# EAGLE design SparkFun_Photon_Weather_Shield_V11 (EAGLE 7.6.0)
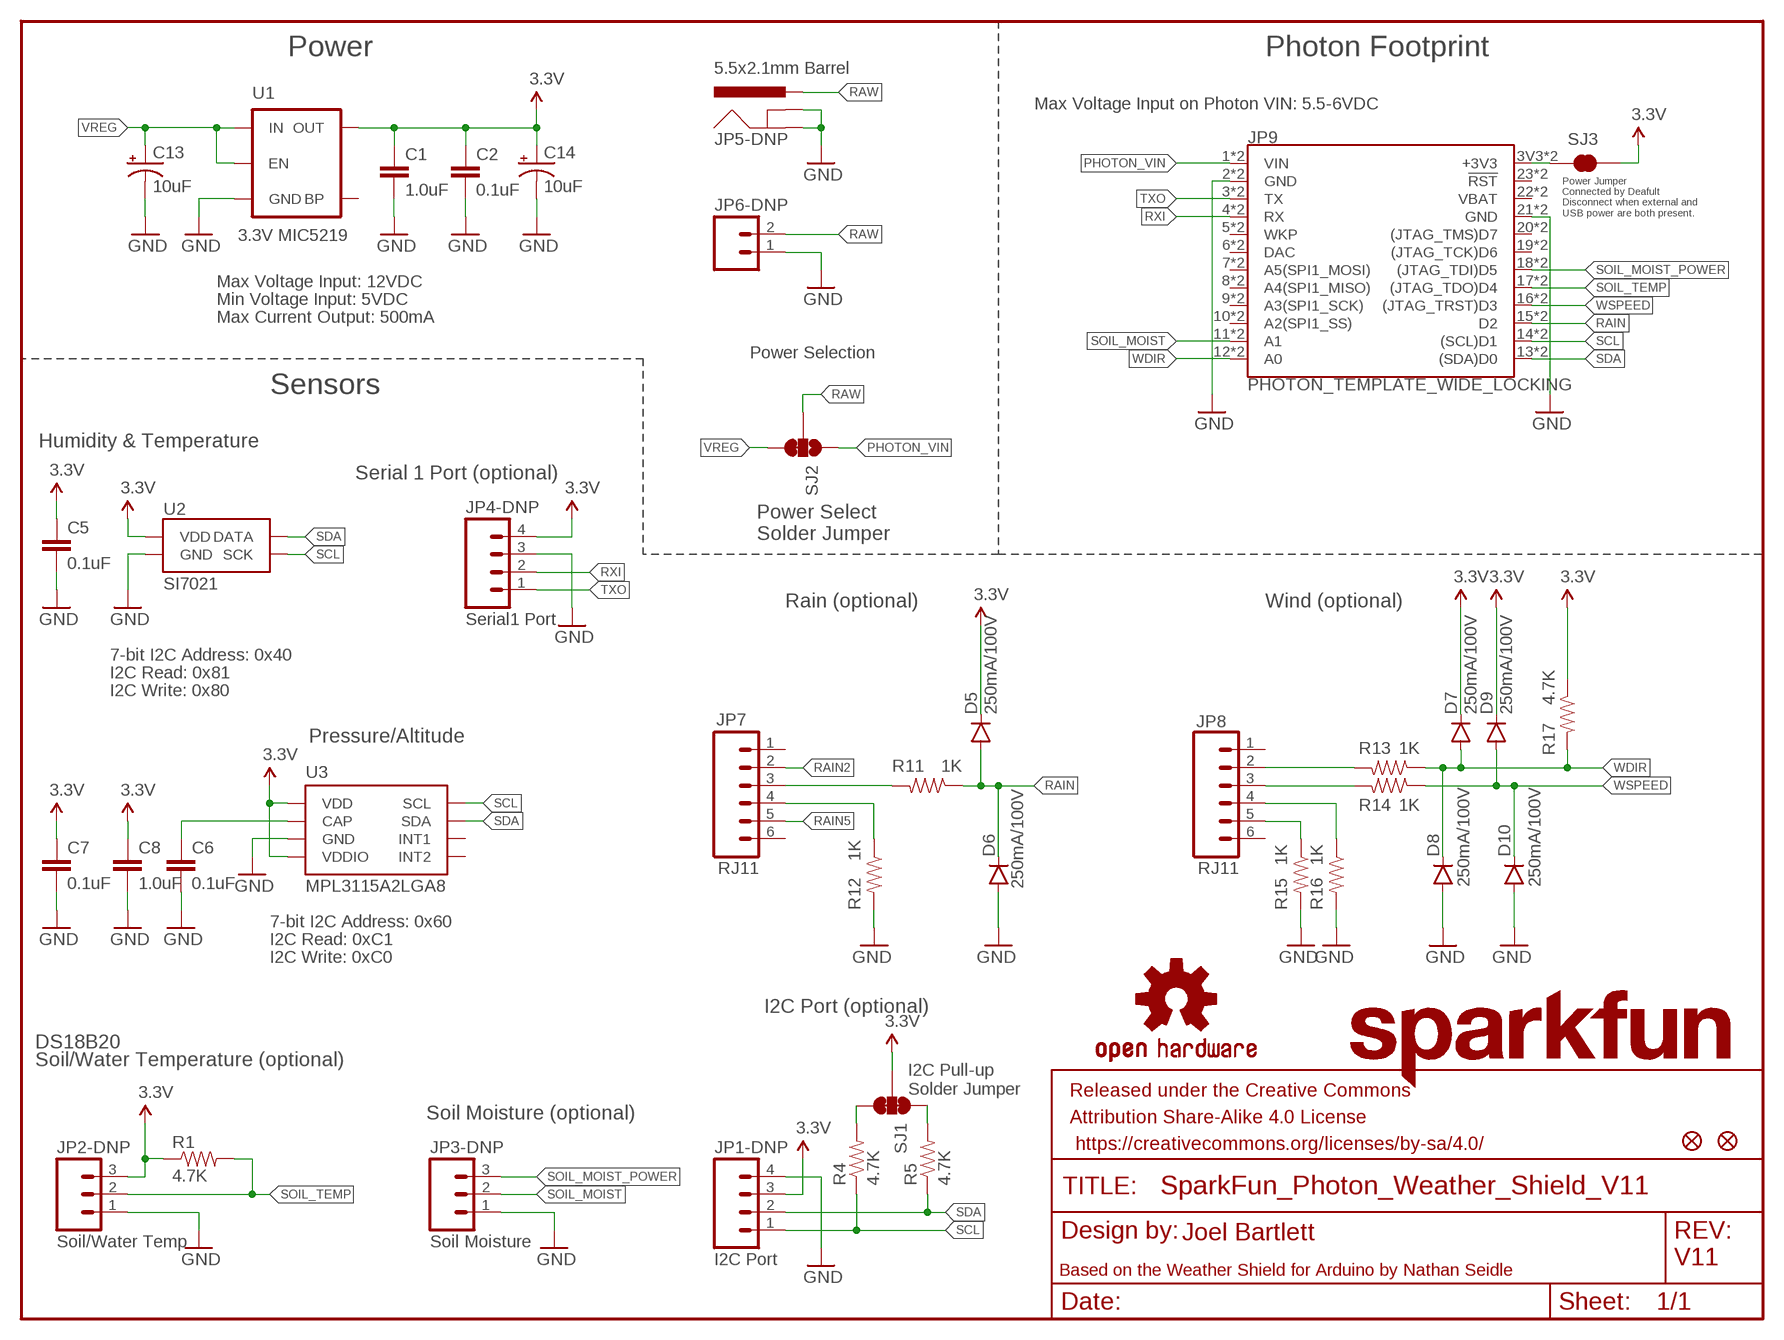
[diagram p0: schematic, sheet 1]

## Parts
C1  1.0uF  1.0UF-16V-10%(0603)  [0603-CAP]
C2  0.1uF  0.1UF-25V(+80/-20%)(0603)  [0603-CAP]
C5  0.1uF  0.1UF-25V(+80/-20%)(0603)  [0603-CAP]
C6  0.1uF  0.1UF-25V(+80/-20%)(0603)  [0603-CAP]
C7  0.1uF  0.1UF-25V(+80/-20%)(0603)  [0603-CAP]
C8  1.0uF  1.0UF-16V-10%(0603)  [0603-CAP]
C13  10uF  10UF-16V-10%(TANT)  [EIA3216]
C14  10uF  10UF-16V-10%(TANT)  [EIA3216]
D5  250mA/100V  DIODEBAS16  [SOD-323]
D6  250mA/100V  DIODEBAS16  [SOD-323]
D7  250mA/100V  DIODEBAS16  [SOD-323]
D8  250mA/100V  DIODEBAS16  [SOD-323]
D9  250mA/100V  DIODEBAS16  [SOD-323]
D10  250mA/100V  DIODEBAS16  [SOD-323]
FID1  FIDUCIAL1X2  [FIDUCIAL-1X2]
FID2  FIDUCIAL1X2  [FIDUCIAL-1X2]
FRAME1  FRAME-LETTER  [CREATIVE_COMMONS]
JP1-DNP  I2C Port  M04PTH  [1X04]
JP2-DNP  Soil/Water Temp  M03PTH  [1X03]
JP3-DNP  Soil Moisture  M03PTH  [1X03]
JP4-DNP  Serial1 Port  M04PTH  [1X04]
JP5-DNP  5.5x2.1mm Barrel  POWER_JACKSMD  [POWER_JACK_SMD]
JP6-DNP  M023.5MM  [SCREWTERMINAL-3.5MM-2]
JP7  RJ11  RJ11-6PTH  [RJ11-6]
JP8  RJ11  RJ11-6PTH  [RJ11-6]
JP9  PHOTON_TEMPLATE_WIDE_LOCKING  SPARK_PHOTONSPARK_PHOTON_TEMPLATE_WIDE_LOCKING  [SPARK_PHOTON_TEMPLATE_WIDE_LOCKING]
LOGO1  OSHW-LOGOM  [OSHW-LOGO-M]
LOGO2  SFE_LOGO_NAME.1_INCH  [SFE_LOGO_NAME_.1]
R1  4.7K  4.7KOHM-1/10W-1%(0603)  [0603-RES]
R4  4.7K  4.7KOHM-1/10W-1%(0603)  [0603-RES]
R5  4.7K  4.7KOHM-1/10W-1%(0603)  [0603-RES]
R11  1K  1KOHM-1/10W-1%(0603)  [0603-RES]
R12  1K  1KOHM-1/10W-1%(0603)  [0603-RES]
R13  1K  1KOHM-1/10W-1%(0603)  [0603-RES]
R14  1K  1KOHM-1/10W-1%(0603)  [0603-RES]
R15  1K  1KOHM-1/10W-1%(0603)  [0603-RES]
R16  1K  1KOHM-1/10W-1%(0603)  [0603-RES]
R17  4.7K  4.7KOHM-1/10W-1%(0603)  [0603-RES]
SJ1  JUMPER-PAD-3-NC_BY_TRACE  [PAD-JUMPER-3-3OF3_NC_BY_TRACE_YES_SILK_FULL_BOX]
SJ2  JUMPER-PAD-3-2OF3_NC_BY_TRACE_SMALL  [PAD-JUMPER-3-2OF3_NC_BY_TRACE_YES_SILK_FULL_BOX]
SJ3  JUMPER-PAD-2-NC_BY_TRACE  [PAD-JUMPER-2-NC_BY_TRACE_YES_SILK]
U1  3.3V MIC5219  MIC52053.3V  [SOT23-5]
U2  SI7021  [SI7021]
U3  MPL3115A2LGA8  [LGA8]

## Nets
3.3V: C1.1 C2.1 C5.1 C7.1 C8.1 C14.A(+) D5.C D7.C D9.C JP1-DNP.3 JP2-DNP.3 JP4-DNP.4 R1.1 R17.1 SJ1.2 SJ3.2 U1.5(OUT) U2.VDD U3.1(VDD) U3.4(VDDIO)
GND: C1.2 C2.2 C5.2 C6.2 C7.2 C8.2 C13.C(-) C14.C(-) D6.A D8.A D10.A JP1-DNP.4 JP2-DNP.1 JP3-DNP.1 JP4-DNP.3 JP5-DNP.GND(GNDBREAK) JP5-DNP.P$4(GND) JP6-DNP.1 JP9.2(GND) JP9.21(GND) JP9.GND@0(GND) JP9.GND@2(GND) R12.2 R15.2 R16.2 U1.2(GND) U2.GND U3.3(GND)
N$1: JP8.3 R14.2
N$2: JP8.2 R13.2
N$3: R4.2 SJ1.3
N$4: JP7.3 R11.2
N$5: C6.1 U3.2(CAP)
N$6: R5.2 SJ1.1
N$7: JP9.3V3(+3V3) JP9.24(+3V3) SJ3.1
N$11: JP7.4 R12.1
N$12: JP8.5 R15.1
N$13: JP8.4 R16.1
PHOTON_VIN: JP9.1(VIN) JP9.VIN SJ2.1
RAIN: D5.A D6.C JP9.15(D2) JP9.D2 R11.1
RAIN2: JP7.2
RAIN5: JP7.5
RAW [vcc]: JP5-DNP.VIN0(PWR) JP6-DNP.2 SJ2.2
RXI: JP4-DNP.2 JP9.4(RX) JP9.RX
SCL: JP1-DNP.1 JP9.14((SCL)D1) JP9.D1((SCL)D1) R4.1 U2.SCK U3.8(SCL)
SDA: JP1-DNP.2 JP9.13((SDA)D0) JP9.D0((SDA)D0) R5.1 U2.DATA U3.7(SDA)
SOIL_MOIST: JP3-DNP.2 JP9.11(A1) JP9.A1
SOIL_MOIST_POWER: JP3-DNP.3 JP9.18((JTAG_TDI)D5) JP9.D5((JTAG_TDI)D5)
SOIL_TEMP: JP2-DNP.2 JP9.17((JTAG_TDO)D4) JP9.D4((JTAG_TDO)D4) R1.2
TXO: JP4-DNP.1 JP9.3(TX) JP9.TX
VREG: C13.A(+) SJ2.3 U1.1(IN) U1.3(EN)
WDIR: D7.A D8.C JP9.12(A0) JP9.A0 R13.1 R17.2
WSPEED: D9.A D10.C JP9.16((JTAG_TRST)D3) JP9.D3((JTAG_TRST)D3) R14.1
Unconnected: JP7.1 JP7.6 JP8.1 JP8.6 JP9.5(WKP) JP9.6(DAC) JP9.7(A5(SPI1_MOSI)) JP9.8(A4(SPI1_MISO)) JP9.9(A3(SPI1_SCK)) JP9.10(A2(SPI1_SS)) JP9.19((JTAG_TCK)D6) JP9.20((JTAG_TMS)D7) JP9.22(VBAT) JP9.23(!RST!) JP9.A2(A2(SPI1_SS)) JP9.A3(A3(SPI1_SCK)) JP9.A4(A4(SPI1_MISO)) JP9.A5(A5(SPI1_MOSI)) JP9.D6((JTAG_TCK)D6) JP9.D7((JTAG_TMS)D7) JP9.DAC JP9.RST(!RST!) JP9.VBAT JP9.WKP U1.4(BP) U3.5(INT2) U3.6(INT1)

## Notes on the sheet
- Power | Photon Footprint
- Max Voltage Input on Photon VIN: 5.5-6VDC
- Power Jumper
  Connected by Deafult
  Disconnect when external and 
  USB power are both present.
- Max Voltage Input: 12VDC
- Min Voltage Input: 5VDC
- Max Current Output: 500mA
- Power Selection
- Sensors
- Humidity & Temperature
- Serial 1 Port (optional)
- Power Select
  Solder Jumper
- Rain (optional) | Wind (optional)
- 7-bit I2C Address: 0x40
- I2C Read: 0x81
- I2C Write: 0x80
- Pressure/Altitude
- 7-bit I2C Address: 0x60
- I2C Read: 0xC1
- I2C Write: 0xC0
- I2C Port (optional)
- DS18B20
- Soil/Water Temperature (optional)
- I2C Pull-up
  Solder Jumper
- Soil Moisture (optional)
- Joel Bartlett
- V11
- Based on the Weather Shield for Arduino by Nathan Seidle

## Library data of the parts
C1 C8 = SparkFun-Capacitors:1.0UF-16V-10%(0603): CAP-00868; PROD_ID: CAP-00868
C2 C5-C7 = SparkFun-Capacitors:0.1UF-25V(+80/-20%)(0603): CAP-00810; PROD_ID: CAP-00810
C13 C14 = SparkFun-Capacitors:10UF-16V-10%(TANT): CAP-00811; PROD_ID: CAP-00811
D5-D10 = SparkFun-DiscreteSemi:DIODE: Diode; PROD_ID: DIO-09646
FID1 FID2 = SparkFun-Aesthetics:FIDUCIAL: Fiducial Alignment Points
FRAME1 = SparkFun-Aesthetics:FRAME-LETTER: Schematic Frame
JP1-DNP JP4-DNP = SparkFun-Connectors:M04: Header 4 Standard 4-pin 0.1" header. Use with straight break away headers (SKU : PRT-00116), right angle break away headers (PRT-00553), swiss pins (PRT-00743), machine pins (PRT-00117), and female headers (PRT-00115). Molex polarized connector foot print use with SKU : PRT-08231 with associated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; PROD_ID: CONN-09696
JP2-DNP JP3-DNP = SparkFun-Connectors:M03: Header 3 Standard 3-pin 0.1" header. Use with straight break away headers (SKU : PRT-00116), right angle break away headers (PRT-00553), swiss pins (PRT-00743), machine pins (PRT-00117), and female headers (PRT-00115). Molex polarized connector foot print use with SKU : PRT-08232 with associated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
JP5-DNP = SparkFun-Connectors:POWER_JACK: Power Jack This is the standard 5.5mm barrel jack for power. The PTH is the most common, proven, reliable, footprint. The Slot footprint only works if the mill layer is transmitted to the PCB fab house so be warned. Mating wall wart : TOL-00298 (and others); PROD_ID: CONN-08106; SF_ID: PRT-12748
JP6-DNP = SparkFun-Connectors:M02: Standard 2-pin 0.1" header. Use with; PROD_ID: CONN-08399
JP7 JP8 = SparkFun-Connectors:RJ11-6: RJ11 Jack Simple 6 pin RJ11 jack. Commonly found on CAT3 devices and Microchip programmers. SKU: PRT-00132; PROD_ID: CONN-08590
JP9 = template_temp:SPARK_PHOTON
LOGO1 = SparkFun-Aesthetics:OSHW-LOGO: Open Source Hardware Logo
LOGO2 = SparkFun-Aesthetics:SFE_LOGO_NAME: SFE Logo, name only
R1 R4 R5 R17 = SparkFun-Resistors:4.7KOHM-1/10W-1%(0603): RES-07857; PROD_ID: RES-07857
R11-R16 = SparkFun-Resistors:1KOHM-1/10W-1%(0603): RES-07856; PROD_ID: RES-07856
SJ1 = SparkFun-Passives:JUMPER-PAD-3-NC_BY_TRACE
SJ2 = SparkFun-Passives:JUMPER-PAD-3-2OF3_NC_BY_TRACE
SJ3 = SparkFun-Passives:JUMPER-PAD-2-NC_BY_TRACE
U1 = SparkFun-PowerIC:MIC5205: MIC5205 150mA vreg 3.3V - VREG-00822 5V - VREG-00823; PROD_ID: VREG-00822
U2 = SparkFun-Sensors:SI7021: The Si7021 is an I2C Humidity and Temperature Sensor; PROD_ID: IC-13093
U3 = SparkFun-Sensors:MPL3115A2: Altimeter/Pressure Sensor, I2C, 1.95V-3.6V supply, 50 to 110kPa; PROD_ID: IC-10869

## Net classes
0 Default: width 0.203 mm
1 vcc: width 0.203 mm

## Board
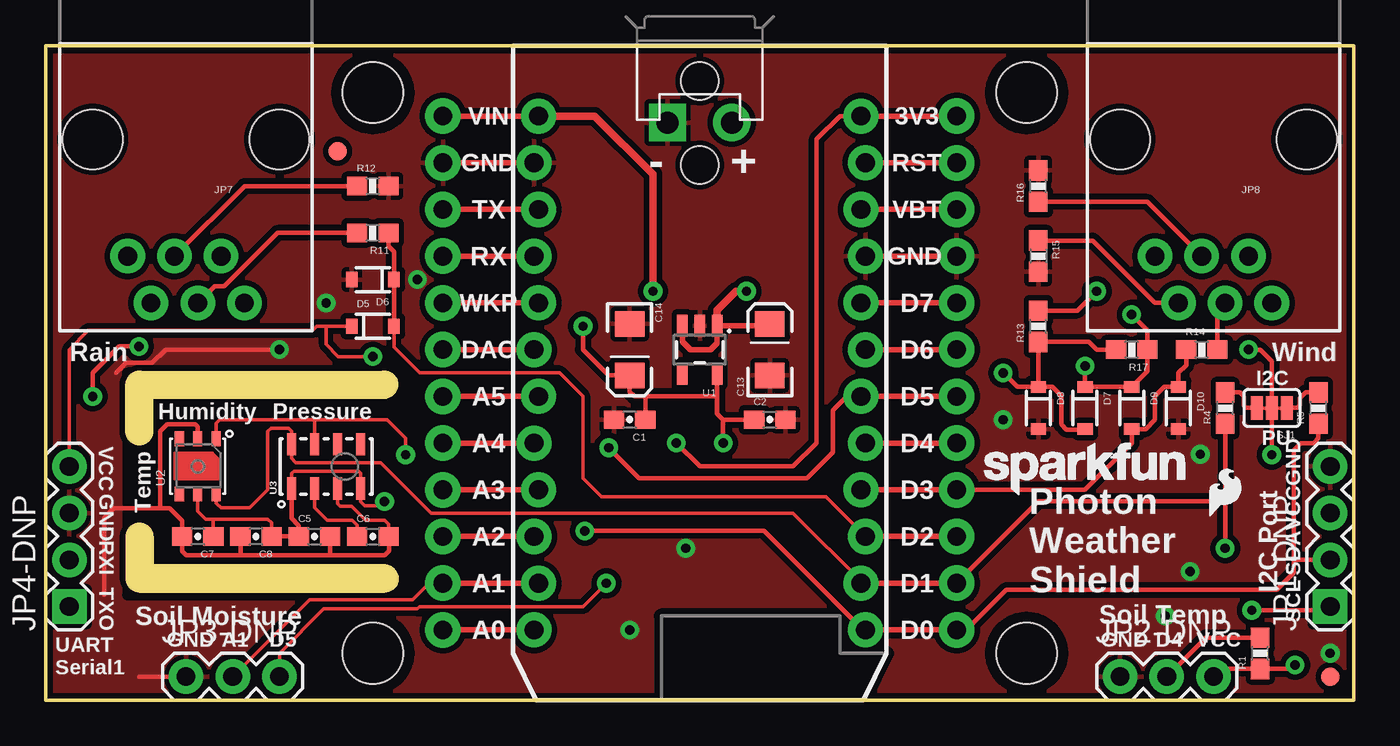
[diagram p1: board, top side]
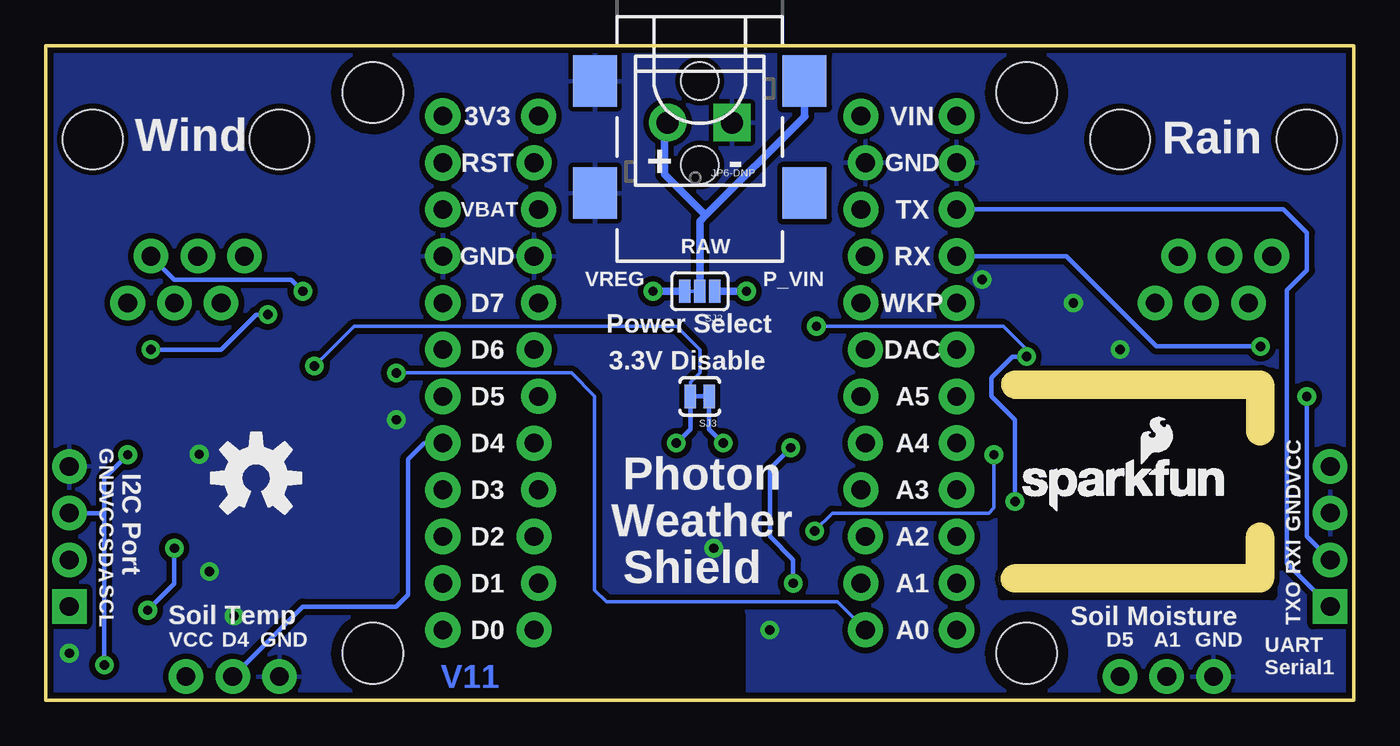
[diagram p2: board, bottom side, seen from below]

Size 71.12 x 35.56 mm. Coordinates in mm from the lower left corner, seen from the top.
Outline: 0,0 0,35.56 71.12,35.56 71.12,0 0,0
Outline: 4.39,17.09 4.39,14.63 arc90 5.08,13.95 arc90 5.74,14.61 5.74,16.46 18.36,16.46 arc90 19.07,17.17 arc90 18.44,17.8 5.11,17.8 arc90 4.39,17.09
Outline: 4.42,6.66 4.42,8.87 arc-90 5.11,9.55 arc-90 5.77,8.87 5.77,7.29 18.39,7.29 arc-90 19.1,6.58 arc-90 18.47,5.94 5.13,5.94 arc-90 4.42,6.66
Copper layers (1*16): Top 0.035mm / dielectric 1.5mm / Bottom 0.035mm
Design rules "SparkFun-2-layer-STANDARD": minimum track width 10mil, minimum drill 20mil, track to track 10mil, track to pad 8mil, pad to pad 8mil, via to via 10mil, smd to smd 8mil, copper to edge 8mil, drill to drill 8mil, minimum pad ring 10mil, minimum via ring 10mil, stop-mask expansion 4mil, vias tented up to drill 25mil, thermal gap 10mil
tRestrict: area 4.4,5.7 to 19.1,17.8
bRestrict: area 4.4,5.7 to 19.1,17.8
Milling: 4 lines

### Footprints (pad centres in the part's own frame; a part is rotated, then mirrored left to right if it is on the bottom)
0603-CAP = smd 1.1 x 1: 1 -0.85,0; 2 0.85,0
EIA3216 = smd 1.4 x 1.6: A 1.4,0; C -1.4,0
SOD-323 = smd 0.63 x 0.83: A 1.15,0; C -1.15,0
FIDUCIAL-1X2 = smd 1 x 1: 1 0,0
1X04 = drill 1.016 pad 1.88 square: 1 0,0 | drill 1.016 pad 1.88: 2 2.54,0; 3 5.08,0; 4 7.62,0
1X03 = drill 1.016 pad 1.88: 1 0,0; 2 2.54,0; 3 5.08,0
POWER_JACK_SMD = smd 2.8 x 2.4: GND 0,-5.7; P$4 6.1,-5.7; VIN0 0,5.7; VIN1 6.1,5.7 | hole 2.032: 0,0; 4.572,0
SCREWTERMINAL-3.5MM-2 = drill 1.2 pad 2.032 square: 1 0,0 | drill 1.2 pad 2.032: 2 3.5,0
RJ11-6 = drill 1.016 pad 1.88: 1 -3.175,8.89; 2 -1.905,6.35; 3 -0.635,8.89; 4 0.635,6.35; 5 1.905,8.89; 6 3.175,6.35 | hole 3.251: -5.08,0; 5.08,0
SPARK_PHOTON_TEMPLATE_WIDE_LOCKING = drill 1.016 pad 1.905: 1 1.397,31.75; 2 1.143,29.21; 3 1.397,26.67; 4 1.143,24.13; 5 1.397,21.59; 6 1.143,19.05; 7 1.397,16.51; 8 1.143,13.97; 9 1.397,11.43; 10 1.143,8.89; 11 1.397,6.35; 12 1.143,3.81; 13 19.177,3.81; 14 18.923,6.35; 15 19.177,8.89; 16 18.923,11.43; 17 19.177,13.97; 18 18.923,16.51; 19 19.177,19.05; 20 18.923,21.59; 21 19.177,24.13; 22 18.923,26.67; 23 19.177,29.21; 24 18.923,31.75 | drill 1.016 pad 1.93: 3V3 24.13,31.75; A0 -3.81,3.81; A1 -3.81,6.35; A2 -3.81,8.89; A3 -3.81,11.43; A4 -3.81,13.97; A5 -3.81,16.51; D0 24.13,3.81; D1 24.13,6.35; D2 24.13,8.89; D3 24.13,11.43; D4 24.13,13.97; D5 24.13,16.51; D6 24.13,19.05; D7 24.13,21.59; DAC -3.81,19.05; GND@0 -3.81,29.21; GND@2 24.13,24.13; RST 24.13,29.21; RX -3.81,24.13; TX -3.81,26.67; VBAT 24.13,26.67; VIN -3.81,31.75; WKP -3.81,21.59 | hole 3.302: -7.62,33.02; 27.94,33.02; -7.62,2.54; 27.94,2.54
0603-RES = smd 1.1 x 1: 1 -0.85,0; 2 0.85,0
PAD-JUMPER-3-3OF3_NC_BY_TRACE_YES_SILK_FULL_BOX = smd 0.635 x 1.27: 1 -0.813,0; 2 0,0; 3 0.813,0
PAD-JUMPER-3-2OF3_NC_BY_TRACE_YES_SILK_FULL_BOX = smd 0.635 x 1.27: 1 -0.813,0; 2 0,0; 3 0.813,0
PAD-JUMPER-2-NC_BY_TRACE_YES_SILK = smd 0.635 x 1.27: 1 -0.508,0; 2 0.508,0
SOT23-5 = smd 0.55 x 1.2: 1 -0.95,-1.3; 2 0,-1.3; 3 0.95,-1.3; 4 0.95,1.3; 5 -0.95,1.3
SI7021 = smd 0.8 x 0.5: DATA 1.5,-1; GND 1.5,0; NC@3 1.5,1; NC@4 -1.5,1; SCK -1.5,-1; VDD -1.5,0
LGA8 = smd 1.2 x 0.5: 1 -1.2,1.875; 2 -1.2,0.625; 3 -1.2,-0.625; 4 -1.2,-1.875; 5 1.2,-1.875; 6 1.2,-0.625; 7 1.2,0.625; 8 1.2,1.875

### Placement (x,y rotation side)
C1  31.75,15.24 180 top
C2  39.37,15.24 0 top
C5  14.61,8.89 0 top
C6  17.78,8.89 0 top
C7  8.26,8.89 180 top
C8  11.43,8.89 180 top
C13  39.37,19.05 90 top
C14  31.75,19.05 270 top
D5  17.78,20.32 0 top
D6  17.78,22.86 180 top
D7  56.52,15.88 270 top
D8  53.98,15.88 270 top
D9  59.05,15.88 270 top
D10  61.59,15.88 270 top
FID1  69.85,1.27 0 top
FID2  15.88,29.84 0 top
FRAME1  not placed on the board
JP1-DNP  69.85,5.08 90 top
JP2-DNP  58.42,1.27 0 top
JP3-DNP  7.62,1.27 0 top
JP4-DNP  1.27,5.08 90 top
JP5-DNP  35.56,33.66 270 bottom
JP6-DNP  33.81,31.39 180 bottom
JP7  7.62,30.48 180 top
JP8  63.5,30.48 180 top
JP9  25.4,0 0 top
LOGO1  59.69,12.06 0 bottom
LOGO2  50.55,10.67 0 top
R1  66.04,2.54 90 top
R4  64.14,15.88 90 top
R5  69.22,15.88 90 top
R11  17.78,25.4 180 top
R12  17.78,27.94 0 top
R13  53.98,20.32 90 top
R14  62.87,19.05 0 top
R15  53.98,24.13 270 top
R16  53.98,27.94 90 top
R17  59.05,19.05 180 top
SJ1  66.67,15.88 180 top
SJ2  35.56,22.23 180 bottom
SJ3  35.56,16.51 180 bottom
U1  35.56,19.05 180 top
U2  8.26,12.7 90 top
U3  15.24,12.7 90 top
U$1  [SFE_LOGO_NAME_FLAME_.1]  18.41,10.19 0 bottom
U$3  [SFE_LOGO_FLAME_.1]  62.99,9.65 0 top

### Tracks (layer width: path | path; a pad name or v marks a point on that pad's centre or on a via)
3.3V  (via drill 0.51)
  Top 0.203: U2.VDD 8.26,10.26 8.69,9.83 9.11,9.83 | 9.11,9.83 12.06,9.83 12.27,9.63 12.27,8.9 C8.1 | 9.11,9.18 9.11,9.83 | U3.1 13.37,12.32 13.49,12.45 16.99,12.45 17.11,12.32 U3.4 | U3.4 | JP4-DNP.4 1.27,19.05 2.31,20.09 14.5,20.09 14.73,20.32 15.24,20.32 | 15.24,20.32 D5.C | v17.78,18.67 15.9,18.67 15.24,19.33 15.24,20.32 | v18.41,10.79 18.19,10.57 17.32,10.57 17.11,10.77 U3.4
  Top 0.254: C7.1 9.11,9.18 | C8.1 C5.1 13.76,9.49 13.37,9.88 U3.1 13.34,11.53 | JP2-DNP.3 63.92,1.69 R1.1 67.73,1.69 v67.94,1.91 | 38.56,15.2 C2.1 36.83,15.24 | v56.52,18.16 D7.C D9.C 59.91,17.88 R17.1 59.91,20.11 v59.05,20.95 | v66.67,13.34 SJ1.2 66.67,18.41 66.04,19.05 v65.41,19.05 | 36.51,16.51 32.6,16.51 | 32.6,16.51 C1.1 | 32.6,16.51 32,16.51 31.75,16.76 C14.A 30.61,17.65 29.21,19.05 v29.21,20.32 | U1.5 36.51,16.51 | 36.51,16.51 36.51,15.56 36.83,15.24 | v36.83,13.97 36.83,15.24 | 17.14,11.47 U3.4
  Bottom 0.203: SJ3.2 36.07,17.27 35.56,17.78 35.56,19.05 36.83,20.32 54.36,20.32 v56.52,18.16 | v29.21,20.32 19.05,20.32 17.78,19.05 v17.78,18.67
  Bottom 0.254: v67.94,1.91 67.94,10.16 | 67.94,10.16 67.94,12.06 v66.67,13.34 | JP1-DNP.3 67.94,10.16 | v65.41,19.05 61.59,19.05 59.69,20.95 v59.05,20.95 | SJ3.2 36.07,14.73 v36.83,13.97 | v18.41,10.79 18.41,15.24 19.68,16.51 19.68,17.53 18.54,18.67 v17.78,18.67
GND  (via drill 0.51)
  Top 0.203: U3.3 15.87,10.68 16,10.54 16.64,10.54 17.4,9.78 18.41,9.78 18.63,9.56 C6.2
  Top 0.254: C6.2 18.67,8.85 18.67,8.13 18.41,7.87 15.46,7.87 | 10.58,7.87 7.62,7.87 7.41,8.09 C7.2 7.41,9.74 6.73,10.41 6.22,10.41 | 10.58,7.87 15.46,7.87 | C5.2 15.46,7.87 | C8.2 10.58,7.87 | 6.22,10.41 3.68,10.41 3.17,9.91 3.17,5.71 | v12.7,19.05 6.5,19.05 5.79,18.34 4.37,18.34 3.81,17.78 | JP3-DNP.1 5.08,1.27 | U2.GND 8.26,14.86 8.13,14.99 6.6,14.99 6.22,14.61 6.22,10.41
  other vias: 52.07,15.24 69.85,2.54 62.79,13.36 60.88,4.57 62.23,6.99 15.24,21.59 20.19,22.86 31.75,3.81 34.8,8.26
  pour Bottom (isolate 0.305): 0,0 0,35.56 71.12,35.56 71.12,0
  pour Top (isolate 0.305): 0,0 0,35.56 71.12,35.56 71.12,0
N$1
  Top 0.254: R14.2 63.72,21.17 JP8.3
N$2  (via drill 0.51)
  Top 0.254: R13.2 56.09,21.17 v57.15,22.23
  Bottom 0.254: JP8.2 64.14,22.86 57.78,22.86 v57.15,22.23
N$3
  Top 0.254: SJ1.3 65.84,15.9 65.25,15.9 65.15,16 65.15,16.51 64.94,16.73 R4.2
N$4
  Top 0.254: JP7.3 9.16,22.5 9.7,22.5 12.6,25.4 R11.2
N$5
  Top 0.203: C6.1 16.93,9.51 16.66,9.78 15.29,9.78 14.62,10.46 U3.2
  Top 0.254: U3.2 14.61,11.49 14.63,11.46
N$6
  Top 0.254: SJ1.1 67.51,15.9 68.07,15.9 68.2,16.03 68.2,16.41 68.52,16.73 R5.2
N$7  (via drill 0.51)
  Top 0.254: v34.29,13.97 35.56,12.7 40.64,12.7 41.91,13.97 41.91,30.48 43.18,31.75 JP9.24 44.45,31.75
  Bottom 0.254: SJ3.1 35.05,14.73 v34.29,13.97
N$11
  Top 0.254: JP7.4 10.79,27.94 R12.1
N$12
  Top 0.254: JP8.5 60.33,21.59 56.94,24.98 R15.1
N$13
  Top 0.254: JP8.4 59.91,27.09 R16.1
PHOTON_VIN  (via drill 0.51)
  Top 0.254: JP9.1 26.67,31.75
  Top 0.406: v33.02,22.23 33.02,28.57 29.84,31.75 JP9.1
  Bottom 0.406: SJ2.1 v33.02,22.23
RAIN
  Top 0.203: D5.A 18.93,19.17 20.32,17.78 27.94,17.78 29.21,16.51 29.21,12.06 30.23,11.05 42.42,11.05 JP9.15 44.45,8.89
  Top 0.254: D5.A D6.C 18.92,24.38 18.63,24.68 R11.1
RAW
  Bottom 0.406: JP6-DNP.2 37.47,31.24 37.47,28.57 35.24,26.35 | JP5-DNP.VIN0 29.86,31.77 29.84,31.75 35.24,26.35 | 35.24,26.35 35.56,26.04 SJ2.2
RXI  (via drill 0.51)
  Top 0.203: JP9.4 26.67,24.13
  Top 0.254: v2.54,16.51 2.54,17.78 3.99,19.23 v5.05,19.23
  Bottom 0.254: JP4-DNP.2 2.54,8.89 v2.54,16.51 | JP9.RX 15.62,24.13 10.72,19.23 v5.05,19.23
SCL  (via drill 0.51)
  Top 0.203: JP9.14 44.45,6.35 40.64,10.16 20.95,10.16 18.21,12.9 13.59,12.9 13.36,13.13 U3.8 13.37,14.63 13.21,14.78 12.24,14.78 12.06,14.61 12.06,11.43 11.07,10.44 9.53,10.44 9.26,10.71 U2.SCK
  Top 0.254: 13.29,13.97 U3.8 | JP1-DNP.1 69.65,4.88 v65.58,4.88 | 64.14,10.79 53.98,10.79 JP9.D1 | v64.14,8.26 64.14,10.79 | R4.1 64.14,10.79
  Bottom 0.254: v64.14,8.26 64.14,6.33 v65.58,4.88
SDA  (via drill 0.51)
  Top 0.203: 14.61,15.24 9.45,15.24 9.25,15.04 9.25,14.21 U2.DATA | 14.61,13.91 14.61,15.24 | 14.61,15.24 18.54,15.24 19.56,14.22 v19.56,13.34
  Top 0.254: 14.61,13.91 U3.7 | JP1-DNP.2 67.87,7.62 | 67.87,7.62 67.87,13.59 68.25,13.97 68.96,13.97 69.22,14.22 R5.1 | 67.87,7.62 67.87,6.91 66.95,5.99 52.25,5.99 50.06,3.81 JP9.D0 | v29.31,9.2 39.04,9.2 44.42,3.81 44.45,3.81 JP9.13
  Bottom 0.203: v29.31,9.2 28.35,10.16 19.84,10.16 19.56,10.44 v19.56,13.34
SOIL_MOIST
  Top 0.203: JP3-DNP.2 14.35,5.46 19.94,5.46 20.83,6.35 JP9.A1 | 26.67,6.35 JP9.11
SOIL_MOIST_POWER  (via drill 0.51)
  Top 0.203: v30.48,6.35 29.21,5.08 20.32,5.08 20.19,4.95 15.11,4.95 12.7,2.54 JP3-DNP.3
  Top 0.254: v30.61,13.72 32.26,12.06 41.4,12.06 42.8,13.46 42.8,15.75 43.56,16.51 JP9.18 44.45,16.51
  Bottom 0.254: v30.61,13.72 31.75,12.57 31.75,8.89 30.48,7.62 v30.48,6.35
SOIL_TEMP
  Top 0.254: R1.2 63.08,3.39 JP2-DNP.2 | JP9.17 44.45,13.97
  Bottom 0.254: JP2-DNP.2 57.15,5.08 52.07,5.08 51.44,5.71 51.44,13.08 50.55,13.97 JP9.D4
TXO
  Top 0.203: 26.67,26.67 JP9.3
  Bottom 0.254: JP4-DNP.1 3.63,7.44 3.63,22.28 2.54,23.37 2.54,25.4 3.81,26.67 JP9.TX
VREG  (via drill 0.51)
  Top 0.305: C13.A 39.27,20.35 U1.1 36.5,19.41 36.14,19.05 35.05,19.05 34.61,19.49 U1.3
  Top 0.406: v38.1,22.23 37.54,22.23 36.5,21.18 U1.1
  Bottom 0.406: SJ2.3 v38.1,22.23
WDIR  (via drill 0.51)
  Top 0.203: JP9.12 26.67,3.81
  Top 0.254: v52.07,17.78 52.83,17.02 D8.C | D7.A 56.5,14.71 55.5,14.71 55.22,14.99 55.22,16.54 54.73,17.02 D8.C | R17.2 57.15,19.05 56.73,19.47 R13.1 D8.C | D8.C
  Bottom 0.203: v52.07,17.78 42.55,17.78 41.27,16.51 41.27,5.97 40.64,5.33 28.07,5.33 JP9.12
WSPEED
  Top 0.203: 44.45,11.43 JP9.16
  Top 0.254: R14.1 62.02,18.2 61.59,17.78 D10.C 60.84,17.02 60.33,16.51 60.33,15.24 59.81,14.72 D9.A 59.05,13.97 56.52,11.43 JP9.D3

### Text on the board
Bottom: V11
Dimension: Route Out | Route Out
tPlace: - | + | Rain | Wind | I2C | Humidity | Pressure | VCC | PU | GND | GND | Temp | RXI | VCC | SDA | TXO | Photon / Weather / Shield | I2C Port | Soil Moisture | Soil Temp | SCL | GND | A1 | D5 | GND | D4 | VCC | UART / Serial1
bPlace: Rain | Wind | - | + | RAW | P_VIN | VREG | Power Select | 3.3V Disable | GND | VCC | I2C Port | Photon | VCC | GND | Weather | SDA | RXI | Shield | SCL | TXO | Soil Moisture | Soil Temp | GND | A1 | D5 | GND | D4 | VCC | UART / Serial1
tDocu: Joel Bartlett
